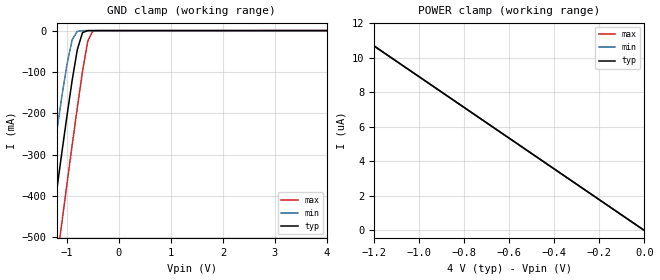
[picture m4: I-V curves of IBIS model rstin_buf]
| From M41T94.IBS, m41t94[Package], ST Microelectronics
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|   Model rstin_buf
[Model]   rstin_buf
Model_type   Input
Vinl =   0.3000V
Vinh =   0.7000V
C_comp   3.2900pF   3.2200pF   4.6400pF
[Temperature Range]   27.0000   85.0000   -40.0000
[Voltage Range]   4.0000V   2.7000V   5.5000V
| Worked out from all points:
|   GND clamp passes 1 mA (typ) near -0.62 V on its own axis
[GND_clamp]
| voltage   I(typ)   I(min)   I(max)
-4V       -3.137A    -2.971A    -3.328A
-1.5V     -676.4mA   -525mA     -855.5mA
-1.4V     -580.3mA   -431.1mA   -757.9mA
-1.3V     -485mA     -338.6mA   -660.7mA
-1.1V     -297.6mA   -161.4mA   -467.6mA
-1V       -207mA     -82.25mA   -372.2mA
-900mV    -120.9mA   -22.43mA   -278.1mA
-800mV    -45.95mA   -1.765mA   -186.1mA
-700mV    -4.783mA   -108.8uA   -98.86mA
-600mV    -164.7uA   -34.13uA   -25.85mA
-500mV    -43.39uA   -29.02uA   -680.4uA
4V        37.72pA    11.58uA    -13.36uA
[POWER_clamp]
| voltage   I(typ)   I(min)   I(max)
-4V       35.63uA    35.63uA    35.63uA
-1.3V     11.58uA    11.58uA    11.58uA
-1.1V     9.797uA    9.797uA    9.797uA
0V        37.72pA    25.67pA    52.3pA
